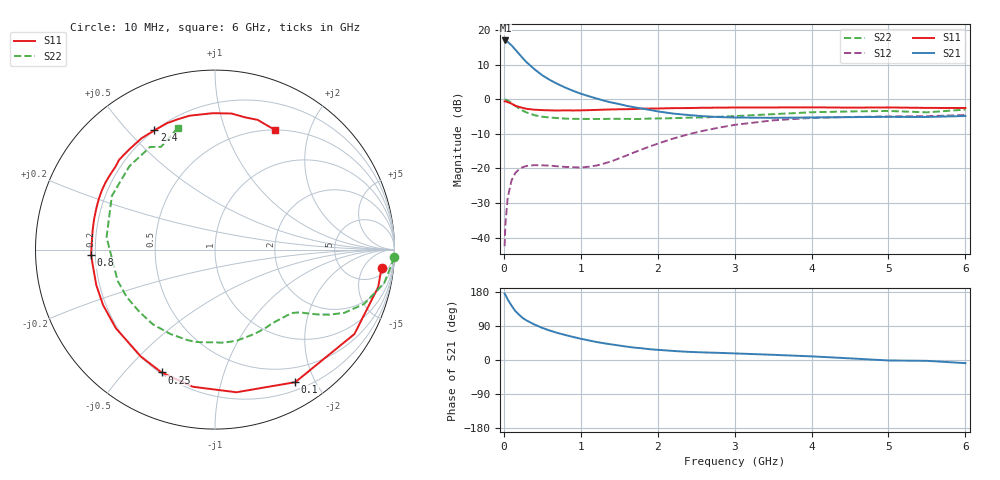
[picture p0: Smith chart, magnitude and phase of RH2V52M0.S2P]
! SIEMENS Small Signal Semiconductors
! BFR106
! Si NPN RF Bipolar Junction Transistor in SOT23
! VCE = 2.5 V  IC = 2 mA
! Common Emitter S-Parameters:  August  1996
# GHz  S  MA  R  50
!  f  S11  S21  S12  S22
! GHz  MAG  ANG  MAG  ANG  MAG  ANG  MAG  ANG
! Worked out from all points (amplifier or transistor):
!   36 points, 10 MHz to 6 GHz, reference 50 ohm
!   highest |S21| = 17.0 dB at 20 MHz (marker M1)
!   |S21| within 3 dB of that: start of sweep to 162.7 MHz
!   unconditionally stable (mu >= 1): 779.1 MHz to 2.098 GHz; 3.378 GHz to end of sweep
!   at 250 MHz: K = 0.32, MSG = 15.7 dB, |S12| = -19.6 dB
!   at 1.4 GHz: K = 1.29, MAG = 5.3 dB, |S12| = -18.0 dB
!   at 6 GHz: K = 1.02, MAG = -1.1 dB, |S12| = -4.6 dB
!   S11 on the Smith chart (normalised r, x): 10 MHz: 8, -13; 100 MHz: 0.30, -1.74; 250 MHz: 0.21, -0.64; 800 MHz: 0.18, -0.02; 2.4 GHz: 0.20, +0.60; 6 GHz: 0.50, +1.50
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0.01  0.9334 -6.3  7.068 175.4  0.0075 87.0  0.9984 -2.5
0.02  0.933 -12.9  7.077 172.0  0.0154 85.2  0.9884 -4.6
0.05  0.9081 -31.2  6.741 159.7  0.0375 73.0  0.9611 -11.1
0.1  0.8635 -58.8  6.012 143.6  0.067 58.6  0.8849 -20.0
0.15  0.8038 -81.5  5.199 129.0  0.086 47.4  0.8014 -26.1
0.2  0.7739 -99.2  4.496 119.0  0.0976 40.1  0.7335 -29.6
0.25  0.7464 -113.5  3.875 110.2  0.1046 34.3  0.6777 -32.2
0.3  0.725 -124.7  3.393 103.8  0.1086 30.8  0.6406 -33.9
0.4  0.705 -141.6  2.705 93.4  0.1114 25.7  0.5867 -36.6
0.5  0.696 -153.6  2.215 84.7  0.1107 23.5  0.5583 -39.2
0.6  0.6904 -163.3  1.894 77.5  0.1096 23.2  0.5441 -42.3
0.8  0.6911 -177.5  1.471 65.9  0.105 26.8  0.5244 -49.5
1.1  0.6951 165.4  1.109 51.8  0.1054 40.6  0.5182 -62.0
1.6  0.7177 144.5  0.8 35.2  0.1543 61.6  0.52 -85.9
2.2  0.7433 123.4  0.62 23.9  0.2696 62.1  0.5319 -117.9
2.4  0.7453 116.9  0.591 21.5  0.3117 59.0  0.5414 -129.8
3  0.7593 100.7  0.544 17.4  0.4255 45.9  0.5696 -162.2
3.5  0.7601 90.9  0.538 13.7  0.4953 34.2  0.608 173.5
4.5  0.7555 77.1  0.551 4.3  0.554 13.6  0.6658 135.8
5  0.7609 71.8  0.556 -1.2  0.5632 5.8  0.6767 122.3
5.5  0.749 66.6  0.554 -2.2  0.5685 2.3  0.6464 117.7
6  0.7467 63.3  0.572 -8.3  0.5911 -5.4  0.7081 107.1
